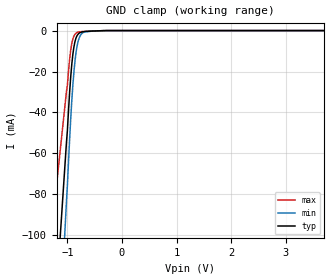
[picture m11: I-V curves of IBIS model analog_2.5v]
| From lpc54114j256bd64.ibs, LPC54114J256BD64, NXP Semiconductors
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[Model] analog_2.5v
Model_type Terminator
C_comp  0.906pF 0.870pF 0.942pF
| variable typ   min   max
[Voltage Range]   2.50000V  2.25000V  2.75000V
[POWER Clamp Reference]  2.50000V  2.25000V  2.75000V
[GND Clamp Reference]   0.00000V  0.00000V  0.00000V
[Temperature Range]   25   85   -40
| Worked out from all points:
|   GND clamp passes 1 mA (typ) near -0.77 V on its own axis
[GND Clamp]
-2.5V     -650.9mA   -842.5mA   -402.9mA
-1.02V    -55.48mA   -84.67mA   -30.29mA
-1V       -48.48mA   -75.13mA   -26.35mA
-960mV    -30.22mA   -53.19mA   -14.04mA
-920mV    -16.39mA   -34.26mA   -6.256mA
-880mV    -7.793mA   -19.86mA   -2.579mA
-860mV    -5.18mA    -14.48mA   -1.702mA
-820mV    -2.307mA   -7.096mA   -882.2uA
-780mV    -1.171mA   -3.277mA   -617.6uA
-740mV    -726.9uA   -1.54mA    -501.3uA
-560mV    -254.6uA   -309.3uA   -218.2uA
5V        0A         0A         0A
[Power Clamp]
-2.5V     0A         0A         0A
0V        0A         0A         0A
2.5V      0A         0A         0A
5V        0A         0A         0A
